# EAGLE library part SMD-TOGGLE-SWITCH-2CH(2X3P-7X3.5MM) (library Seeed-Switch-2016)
311030005
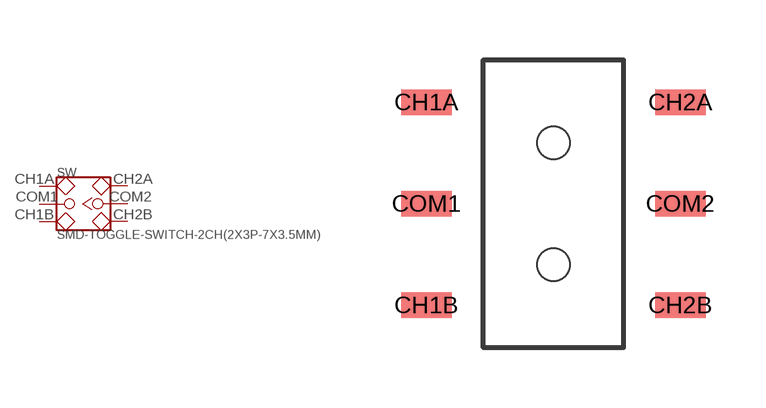
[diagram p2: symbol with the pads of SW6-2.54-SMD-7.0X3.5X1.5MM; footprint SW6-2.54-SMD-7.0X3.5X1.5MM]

Designator prefix SW

## SMD-TOGGLE-SWITCH-2CH(2X3P-7X3.5MM)  [SW6-2.54-SMD-7.0X3.5X1.5MM]
CH1A  CH1A
CH1B  CH1B
CH2A  CH2A
CH2B  CH2B
COM1  COM1
COM2  COM2

## Footprint SW6-2.54-SMD-7.0X3.5X1.5MM (pad centres in mm)
smd 1.27 x 0.635: CH1A -3.175,2.54; CH1B -3.175,-2.54; CH2A 3.175,2.54; CH2B 3.175,-2.54; COM1 -3.175,0; COM2 3.175,0
hole 0.813 at 0,1.524
hole 0.813 at 0,-1.524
